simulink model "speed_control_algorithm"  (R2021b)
settings: Solver=FixedStepDiscrete  StartTime=0.0  StopTime=10.0  RelTol=1e-3
InitFcn:
  | foc_qep_data;
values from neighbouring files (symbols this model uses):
  PI_params = mcb.internal.SetControllerParameters(pmsm,inverter,PU_System,T_pwm,5*Ts,Ts_speed)    [foc_qep_data.m]
  Ts = T_pwm    (= 5e-05)    [foc_qep_data.m]    (also in open_loop_data.m; qep_calibration_data.m)
  Ts_speed = 10*Ts    (= 0.0005)    [foc_qep_data.m]
libraries: mcbcontrolslib x2

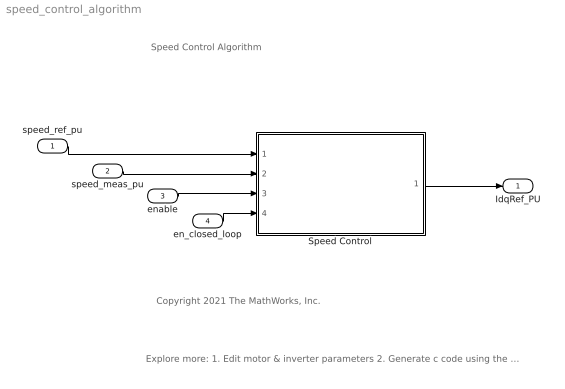
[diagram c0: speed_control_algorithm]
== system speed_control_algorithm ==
  note: Speed Control Algorithm
  note: Explore more: 1. Edit motor & inverter parameters 2. Generate c code using the 'Embedded Coder' app 3. Integrate generated code with driver code 4. Control motor via host model
  note: Copyright 2021 The MathWorks, Inc.
  speed_ref_pu : Inport  OutDataTypeStr=dataType
  speed_meas_pu : Inport  Port=2  OutDataTypeStr=dataType
  enable : Inport  Port=3  OutDataTypeStr=boolean
  en_closed_loop : Inport  Port=4  OutDataTypeStr=boolean
  Speed Control : Subsystem  TreatAsAtomicUnit=on  SystemSampleTime=Ts_speed
  IdqRef_PU : Outport  OutDataTypeStr=dataType  PortDimensions=2
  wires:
  speed_ref_pu/1 -> Speed Control/1(Speed_Ref_PU)
  speed_meas_pu/1 -> Speed Control/2(Speed_Meas_PU)
  enable/1 -> Speed Control/3(enable)
  en_closed_loop/1 -> Speed Control/4(en_closed_loop)
  Speed Control/1(IdqRef_PU) -> IdqRef_PU/1

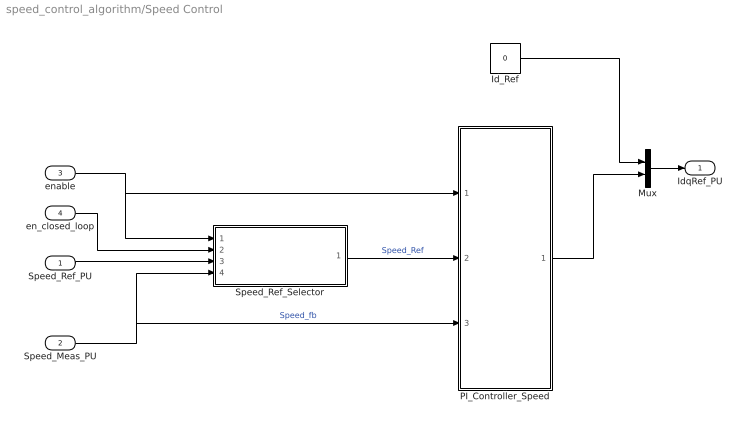
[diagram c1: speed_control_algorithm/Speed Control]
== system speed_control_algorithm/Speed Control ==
  Speed_Ref_PU : Inport
  Speed_Meas_PU : Inport  Port=2
  enable : Inport  Port=3
  en_closed_loop : Inport  Port=4
  Id_Ref : Constant  Value=0  OutDataTypeStr=dataType
  Mux : Mux  Inputs=2
  PI_Controller_Speed : Subsystem
  Speed_Ref_Selector : Subsystem
  IdqRef_PU : Outport  VectorParamsAs1DForOutWhenUnconnected=off
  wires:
  PI_Controller_Speed/1(Iq_ref) -> Mux/2
  Speed_Meas_PU/1 -> Speed_Ref_Selector/4(Speed_Ref_Open), PI_Controller_Speed/3(N_fb)  "Speed_fb"
  Id_Ref/1 -> Mux/1
  Mux/1 -> IdqRef_PU/1
  Speed_Ref_Selector/1(Speed_Ref_PU) -> PI_Controller_Speed/2(N_ref)  "Speed_Ref"
  enable/1 -> Speed_Ref_Selector/1(enable), PI_Controller_Speed/1(enable)
  en_closed_loop/1 -> Speed_Ref_Selector/2(en_closed_loop)
  Speed_Ref_PU/1 -> Speed_Ref_Selector/3(Speed_Ref_In)

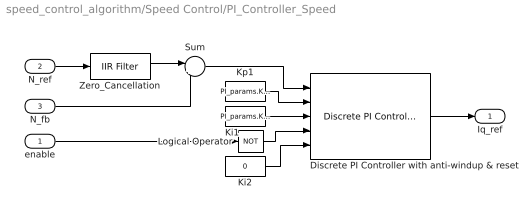
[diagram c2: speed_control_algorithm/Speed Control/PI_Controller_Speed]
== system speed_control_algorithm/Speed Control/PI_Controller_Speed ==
  enable : Inport
  N_ref : Inport  Port=2
  N_fb : Inport  Port=3
  Discrete PI Controller with anti-windup & reset : mcbcontrolslib/Discrete PI Controller  with anti-windup & reset  UpperSaturationLimit=1  LowerSaturationLimit=-1
  Ki1 : Constant  Value=PI_params.Ki_speed*Ts_speed  OutDataTypeStr=dataType  SampleTime=-1
  Ki2 : Constant  Value=0  OutDataTypeStr=dataType  SampleTime=-1
  Kp1 : Constant  Value=PI_params.Kp_speed  OutDataTypeStr=dataType  SampleTime=-1
  Logical Operator : Logic  Operator=NOT  IconShape=distinctive  AllPortsSameDT=off  OutDataTypeStr=boolean
  Sum : Sum  Inputs=|+-
  Zero_Cancellation : mcbcontrolslib/IIR Filter  VariantControl=Low Pass Filter  VariantSelect=Low-pass  Filter_constant=0.01*(Ts_speed/Ts)  advancedSettings=off  Ts=50e-6  cutOff_freq=1
  Iq_ref : Outport  VectorParamsAs1DForOutWhenUnconnected=off
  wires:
  Discrete PI Controller with anti-windup & reset/1 -> Iq_ref/1
  Ki1/1 -> Discrete PI Controller with anti-windup & reset/3
  Kp1/1 -> Discrete PI Controller with anti-windup & reset/2
  N_fb/1 -> Sum/2
  N_ref/1 -> Zero_Cancellation/1
  Sum/1 -> Discrete PI Controller with anti-windup & reset/1
  Logical Operator/1 -> Discrete PI Controller with anti-windup & reset/4
  Ki2/1 -> Discrete PI Controller with anti-windup & reset/5
  enable/1 -> Logical Operator/1
  Zero_Cancellation/1 -> Sum/1

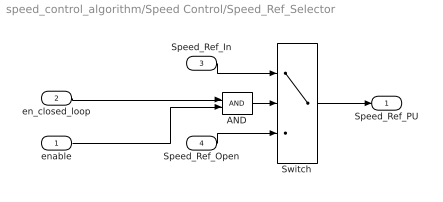
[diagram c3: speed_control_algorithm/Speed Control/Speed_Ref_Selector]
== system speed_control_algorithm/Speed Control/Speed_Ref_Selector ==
  enable : Inport
  en_closed_loop : Inport  Port=2
  Speed_Ref_In : Inport  Port=3
  Speed_Ref_Open : Inport  Port=4
  AND : Logic  IconShape=distinctive  AllPortsSameDT=off  OutDataTypeStr=boolean
  Switch : Switch  Criteria=u2 > Threshold  Threshold=0.5
  Speed_Ref_PU : Outport
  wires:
  Switch/1 -> Speed_Ref_PU/1
  Speed_Ref_Open/1 -> Switch/3
  Speed_Ref_In/1 -> Switch/1
  AND/1 -> Switch/2
  en_closed_loop/1 -> AND/1
  enable/1 -> AND/2
